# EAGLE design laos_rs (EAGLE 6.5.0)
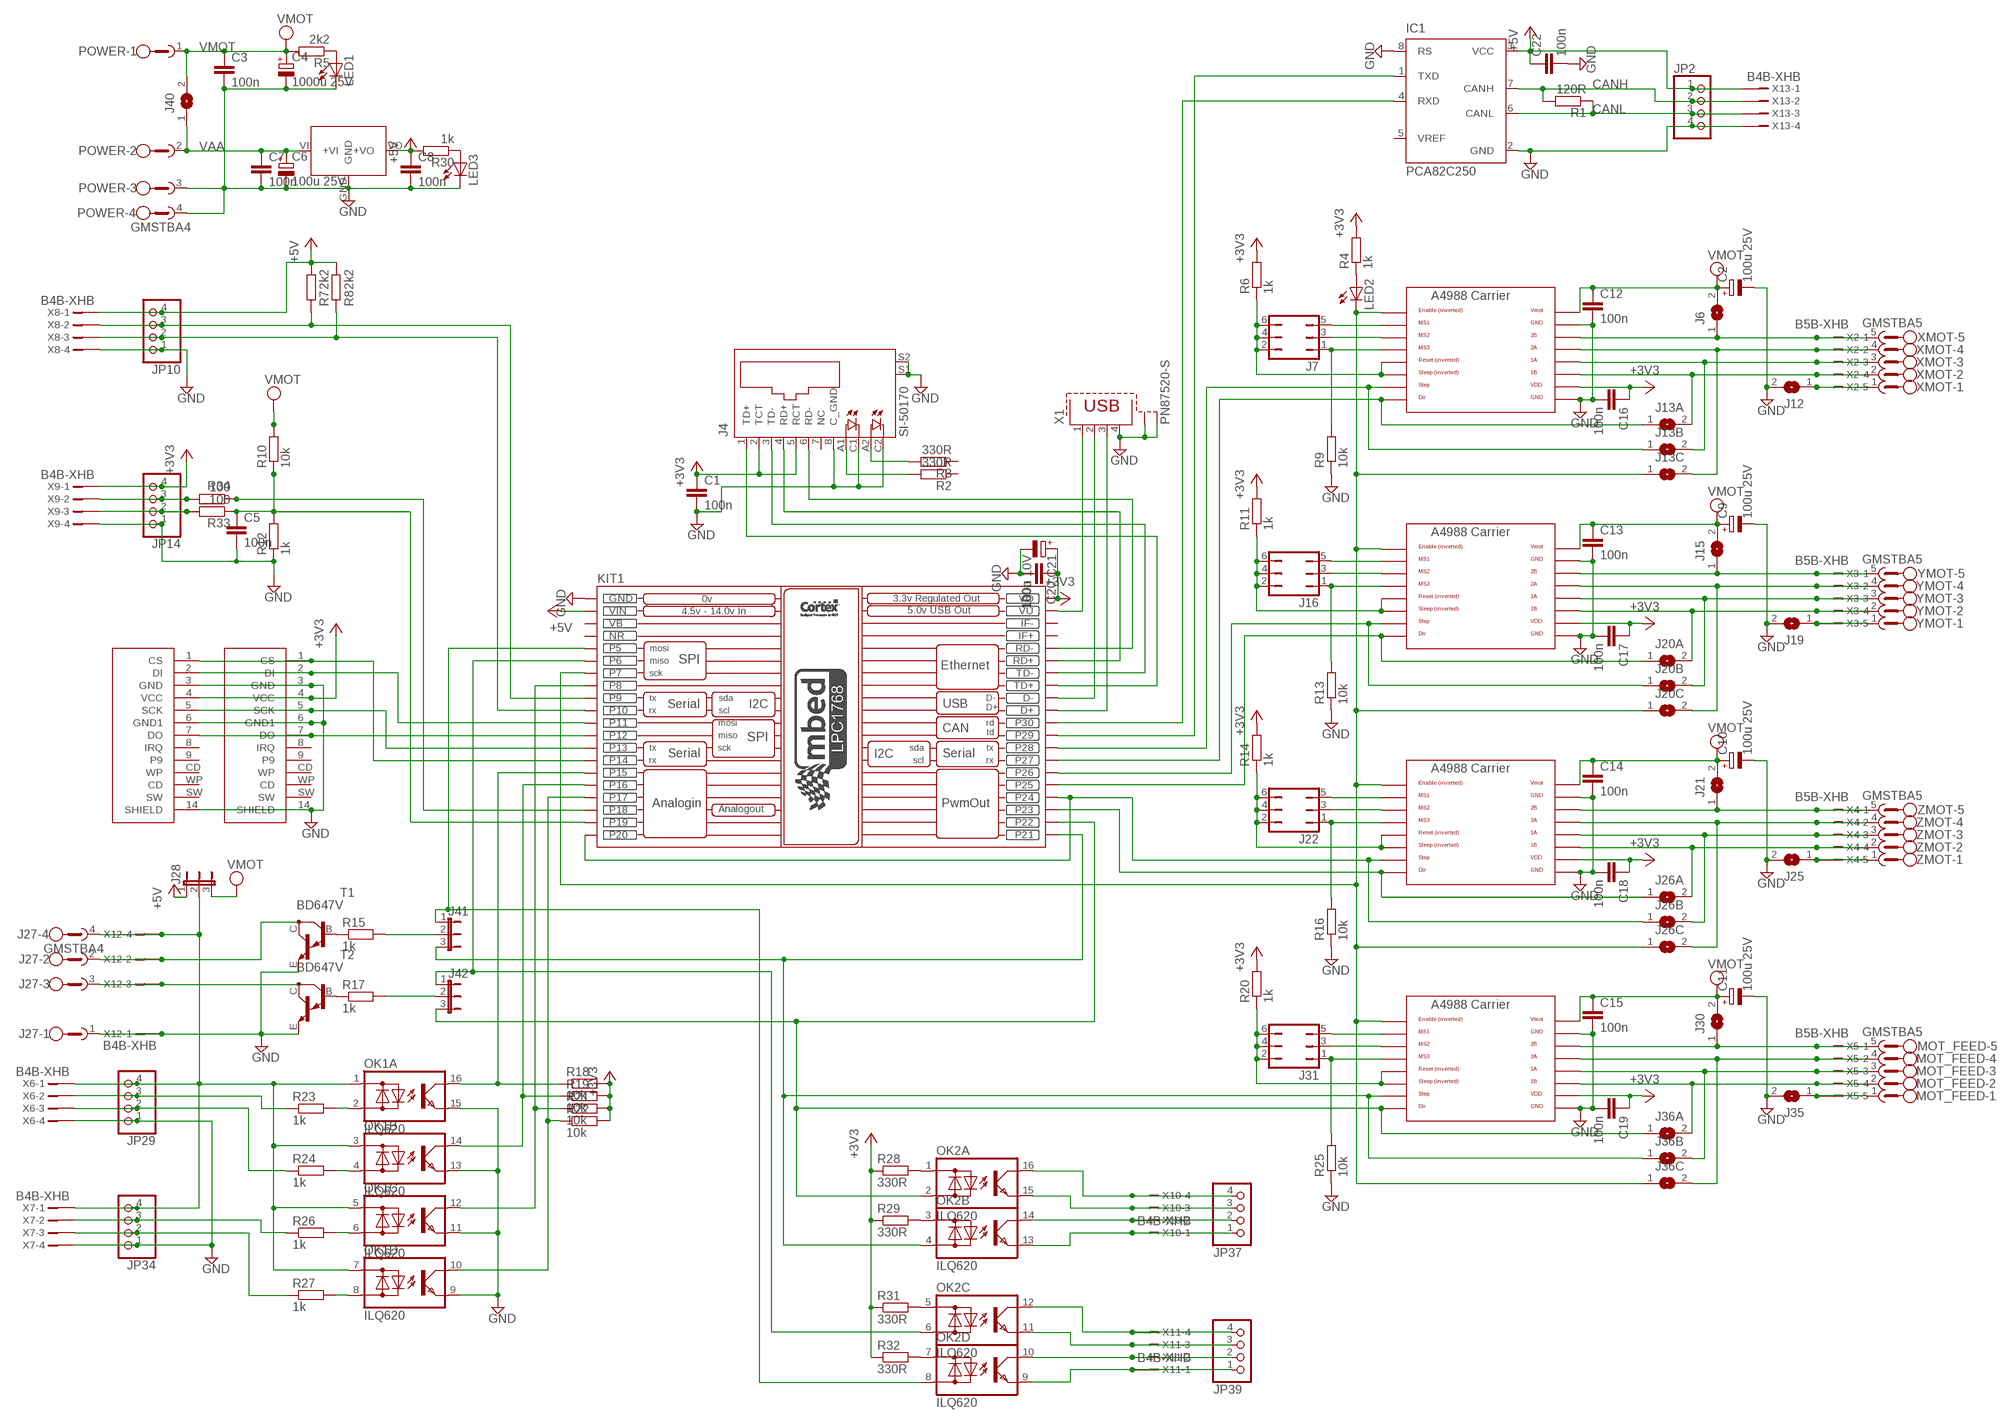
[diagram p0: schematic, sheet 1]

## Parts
C1  100n  C-EU025_050-025X075  [C025_050-025X075]
C2  100u 25V  CPOL-EUE5-8.5  [E5-8,5]
C3  100n  C-EU025_050-025X075  [C025_050-025X075]
C4  1000u 25V  CPOL-EUE5-13  [E5-13]
C5  100n  C-EU050-025X075  [C050-025X075]
C6  100u 25V  CPOL-EUE5-10.5  [E5-10,5]
C7  100n  C-EU025_050-025X075  [C025_050-025X075]
C8  100n  C-EU025_050-025X075  [C025_050-025X075]
C9  100u 25V  CPOL-EUE5-8.5  [E5-8,5]
C10  100u 25V  CPOL-EUE5-8.5  [E5-8,5]
C11  100u 25V  CPOL-EUE5-8.5  [E5-8,5]
C12  100n  C-EU025_050-025X075  [C025_050-025X075]
C13  100n  C-EU025_050-025X075  [C025_050-025X075]
C14  100n  C-EU025_050-025X075  [C025_050-025X075]
C15  100n  C-EU025_050-025X075  [C025_050-025X075]
C16  100n  C-EU025_050-025X075  [C025_050-025X075]
C17  100n  C-EU025_050-025X075  [C025_050-025X075]
C18  100n  C-EU025_050-025X075  [C025_050-025X075]
C19  100n  C-EU025_050-025X075  [C025_050-025X075]
C20  100n  C-EU025_050-025X075  [C025_050-025X075]
C21  100u 10V  CPOL-EUE5-8.5  [E5-8,5]
C22  100n  C-EU025_050-025X075  [C025_050-025X075]
IC1  PCA82C250  [DIL08]
J4  SI-50170  [SI-50170]
J6  SJ  [SJ]
J7  JP3Q  [JP3Q]
J12  SJ  [SJ]
J13A  SJ  [SJ]
J13B  SJ  [SJ]
J13C  SJ  [SJ]
J15  SJ  [SJ]
J16  JP3Q  [JP3Q]
J19  SJ  [SJ]
J20A  SJ  [SJ]
J20B  SJ  [SJ]
J20C  SJ  [SJ]
J21  SJ  [SJ]
J22  JP3Q  [JP3Q]
J25  SJ  [SJ]
J26A  SJ  [SJ]
J26B  SJ  [SJ]
J26C  SJ  [SJ]
J27  GMSTBA4  [GMSTBA4]
J28  JP2E  [JP2]
J30  SJ  [SJ]
J31  JP3Q  [JP3Q]
J35  SJ  [SJ]
J36A  SJ  [SJ]
J36B  SJ  [SJ]
J36C  SJ  [SJ]
J40  SJW  [SJW]
J41  JP2E  [JP2]
J42  JP2E  [JP2]
JP2  PINHD-1X04_2.54  [1X04]
JP10  PINHD-1X04_2.54  [1X04]
JP14  PINHD-1X04_2.54  [1X04]
JP29  PINHD-1X04_2.54  [1X04]
JP34  PINHD-1X04_2.54  [1X04]
JP37  PINHD-1X04_2.54  [1X04]
JP39  PINHD-1X04_2.54  [1X04]
KIT1  MBED_NXP_LPC1768  [MBED-KIT]
LED1  LED3MM  [LED3MM]
LED2  LED3MM  [LED3MM]
LED3  LED3MM  [LED3MM]
MOT_FEED  GMSTBA5  [GMSTBA5]
OK1  ILQ620  [DIL16]
OK2  ILQ620  [DIL16]
POWER  GMSTBA4  [GMSTBA4]
R1  120R  R-EU0207/2V  [0207/2V]
R2  330R  R-EU0207/10  [0207/10]
R3  330R  R-EU0207/10  [0207/10]
R4  1k  R-EU0207/10  [0207/10]
R5  2k2  R-EU0207/10  [0207/10]
R6  1k  R-EU0207/10  [0207/10]
R7  2k2  R-EU0207/10  [0207/10]
R8  2k2  R-EU0207/10  [0207/10]
R9  10k  R-EU0207/10  [0207/10]
R10  10k  R-EU0207/10  [0207/10]
R11  1k  R-EU0207/10  [0207/10]
R12  1k  R-EU0207/10  [0207/10]
R13  10k  R-EU0207/10  [0207/10]
R14  1k  R-EU0207/10  [0207/10]
R15  1k  R-EU0207/10  [0207/10]
R16  10k  R-EU0207/10  [0207/10]
R17  1k  R-EU0207/10  [0207/10]
R18  10k  R-EU0207/10  [0207/10]
R19  10k  R-EU0207/10  [0207/10]
R20  1k  R-EU0207/10  [0207/10]
R21  10k  R-EU0207/10  [0207/10]
R22  10k  R-EU0207/10  [0207/10]
R23  1k  R-EU0207/10  [0207/10]
R24  1k  R-EU0207/10  [0207/10]
R25  10k  R-EU0207/10  [0207/10]
R26  1k  R-EU0207/10  [0207/10]
R27  1k  R-EU0207/10  [0207/10]
R28  330R  R-EU0207/10  [0207/10]
R29  330R  R-EU0207/10  [0207/10]
R30  1k  R-EU0207/10  [0207/10]
R31  330R  R-EU0207/10  [0207/10]
R32  330R  R-EU0207/10  [0207/10]
R33  100  R-EU0207/10  [0207/10]
R34  100  R-EU0207/10  [0207/10]
T1  BD647V  [TO220AV]
T2  BD647V  [TO220AV]
U4  SD_CARD_SOCKETSD  [SD-MMC_SOCKET-PP]
U11  SD_CARD_SOCKETSD  [SD-MMC_SOCKET-PP]
U$1  POLOLU_A4983CARRIER  [A4988BREAKOUT]
U$2  POLOLU_A4983CARRIER  [A4988BREAKOUT]
U$3  POLOLU_A4983CARRIER  [A4988BREAKOUT]
U$5  R-78B-  [R-78B**-*]
U$6  POLOLU_A4983CARRIER  [A4988BREAKOUT]
X1  PN87520-S  [PN87520-S]
X2  B5B-XHB  [B5B-XH]
X3  B5B-XHB  [B5B-XH]
X4  B5B-XHB  [B5B-XH]
X5  B5B-XHB  [B5B-XH]
X6  B4B-XHB  [B4B-XH]
X7  B4B-XHB  [B4B-XH]
X8  B4B-XHB  [B4B-XH]
X9  B4B-XHB  [B4B-XH]
X10  B4B-XHB  [B4B-XH]
X11  B4B-XHB  [B4B-XH]
X12  B4B-XHB  [B4B-XH]
X13  B4B-XHB  [B4B-XH]
XMOT  GMSTBA5  [GMSTBA5]
YMOT  GMSTBA5  [GMSTBA5]
ZMOT  GMSTBA5  [GMSTBA5]

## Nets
+3V3: C1.1 C16.1 C17.1 C18.1 C19.1 C20.1 C21.+ J4.2(TCT) J4.5(RCT) JP14.4 KIT1.VOUT(VO) R4.2 R6.2 R11.2 R14.2 R18.2 R19.2 R20.2 R21.2 R22.2 R28.1 R29.1 R31.1 R32.1 U4.4(VCC) U11.4(VCC) U$1.VDD U$2.VDD U$3.VDD U$6.VDD X9.1
+5V: C8.1 C22.1 IC1.3(VCC) J28.1 JP2.1 JP10.4 KIT1.VIN R7.2 R8.2 R30.2 U$5.VO(+VO) X8.1 X13.1
/ENABLE: J13C.1 J20C.1 J26C.1 J36C.1 KIT1.7 LED2.K(C) U$1.EN U$2.EN U$3.EN U$6.EN
ANALOG_IN: C5.1 KIT1.19 R10.1 R12.2 R33.1
ANALOG_OUT: KIT1.18 R34.1
AUX1: J27.2 T1.C X12.2
AUX2: J27.3 T2.C X12.3
CANH: IC1.7(CANH) JP2.2 R1.2 X13.2
CANL: IC1.6(CANL) JP2.3 R1.1 X13.3
D+: KIT1.D+ X1.3
D-: KIT1.D- X1.2
DIR_FEED: J36A.1 J42.3 KIT1.22 OK2.2(A:AC2) U$6.DIR
DIR_X: J13A.1 KIT1.27 U$1.DIR
DIR_Y: J20A.1 KIT1.25 U$2.DIR
DIR_Z: J26A.1 KIT1.23 U$3.DIR
EXHAUST_ENABLE_C: JP37.4 OK2.16(A:C) X10.4
EXHAUST_ENABLE_E: JP37.3 OK2.15(A:E) X10.3
GND: C1.2 C1.3 C2.- C3.2 C3.3 C4.- C5.2 C6.- C7.2 C7.3 C8.2 C8.3 C9.- C10.- C11.- C12.2 C12.3 C13.2 C13.3 C14.2 C14.3 C15.2 C15.3 C16.2 C16.3 C17.2 C17.3 C18.2 C18.3 C19.2 C19.3 C20.2 C20.3 C21.- C22.2 C22.3 IC1.2(GND) IC1.8(RS) J4.8(C_GND) J4.C1(C) J4.C2(C1) J4.S1 J4.S2 J12.2 J19.2 J25.2 J27.1 J35.2 JP2.4 JP10.1 JP14.1 JP29.1 JP34.1 KIT1.GND LED1.K(C) LED3.K(C) OK1.9(D:E) OK1.11(C:E) OK1.13(B:E) OK1.15(A:E) POWER.3 POWER.4 R9.1 R12.1 R13.1 R16.1 R25.1 T1.E T2.E U4.3(GND) U4.6(GND1) U4.14(SHIELD) U11.3(GND) U11.6(GND1) U11.14(SHIELD) U$1.GND U$1.GND@0(GND) U$2.GND U$2.GND@0(GND) U$3.GND U$3.GND@0(GND) U$5.GND U$6.GND U$6.GND@0(GND) X1.4 X1.S1 X1.S2 X6.4 X7.4 X8.4 X9.4 X12.1 X13.4
LASER_ENABLE_C: JP37.2 OK2.14(B:C) X10.2
LASER_ENABLE_E: JP37.1 OK2.13(B:E) X10.1
LASER_ON: J41.1 KIT1.5 OK2.8(D:AC2)
LASER_ON_E: JP39.1 OK2.9(D:E) X11.1
LASER_PWM: J42.1 KIT1.6 OK2.6(C:AC2)
LASER_PWM_C: JP39.4 OK2.12(C:C) X11.4
LASER_PWM_E: JP39.3 OK2.11(C:E) X11.3
N$1: J15.1 U$2.2B X3.1 YMOT.5
N$2: J20C.2 U$2.2A X3.2 YMOT.4
N$3: J20B.2 U$2.1A X3.3 YMOT.3
N$4: J20A.2 U$2.1B X3.4 YMOT.2
N$5: J6.1 U$1.2B X2.1 XMOT.5
N$6: J13C.2 U$1.2A X2.2 XMOT.4
N$7: J13B.2 U$1.1A X2.3 XMOT.3
N$8: J13A.2 U$1.1B X2.4 XMOT.2
N$9: J21.1 U$3.2B X4.1 ZMOT.5
N$10: J26C.2 U$3.2A X4.2 ZMOT.4
N$11: J26B.2 U$3.1A X4.3 ZMOT.3
N$12: J26A.2 U$3.1B X4.4 ZMOT.2
N$13: OK2.1(A:AC1) R28.2
N$14: OK2.3(B:AC1) R29.2
N$15: OK2.5(C:AC1) R31.2
N$16: OK2.7(D:AC1) R32.2
N$17: OK1.2(A:AC2) R23.2
N$18: OK1.4(B:AC2) R24.2
N$19: OK1.6(C:AC2) R26.2
N$20: OK1.8(D:AC2) R27.2
N$22: J12.1 X2.5 XMOT.1
N$23: J19.1 X3.5 YMOT.1
N$24: J25.1 X4.5 ZMOT.1
N$28: KIT1.VU X1.1
N$29: J7.2 J7.4 J7.6 R6.1 U$1.RST U$1.SLP(SLEEP)
N$30: J7.5 U$1.MS1
N$31: J7.3 U$1.MS2
N$32: J7.1 R9.2 U$1.MS3
N$34: J16.2 J16.4 J16.6 R11.1 U$2.RST U$2.SLP(SLEEP)
N$35: J16.5 U$2.MS1
N$36: J16.3 U$2.MS2
N$37: J16.1 R13.2 U$2.MS3
N$39: J22.2 J22.4 J22.6 R14.1 U$3.RST U$3.SLP(SLEEP)
N$40: J22.5 U$3.MS1
N$41: J22.3 U$3.MS2
N$42: J22.1 R16.2 U$3.MS3
N$49: JP14.2 R33.2 X9.3
N$55: J35.1 MOT_FEED.1 X5.5
N$57: J4.A1(A) R2.2
N$60: JP14.3 R34.2 X9.2
N$64: R15.1 T1.B
N$65: R17.1 T2.B
N$68: JP39.2 OK2.10(D:C) X11.2
N$75: J4.A2(A1) R3.2
N$76: J41.2 R15.2
N$77: J42.2 R17.2
N$82: J30.1 MOT_FEED.5 U$6.2B X5.1
N$83: J36C.2 MOT_FEED.4 U$6.2A X5.2
N$84: J36B.2 MOT_FEED.3 U$6.1A X5.3
N$85: J36A.2 MOT_FEED.2 U$6.1B X5.4
N$86: LED3.A R30.1
N$90: J31.2 J31.4 J31.6 R20.1 U$6.RST U$6.SLP(SLEEP)
N$91: J31.5 U$6.MS1
N$92: J31.3 U$6.MS2
N$93: J31.1 R25.2 U$6.MS3
N$105: LED1.A R5.1
N$106: LED2.A R4.1
P8: KIT1.8 OK1.12(C:C) R21.1
P11: KIT1.11 U4.2(DI) U11.2(DI)
P12: KIT1.12 U4.7(DO) U11.7(DO)
P13: KIT1.13 U4.5(SCK) U11.5(SCK)
P14: KIT1.14 U4.1(CS) U11.1(CS)
P15: KIT1.15 OK1.16(A:C) R18.1
P16: KIT1.16 OK1.14(B:C) R19.1
P17: KIT1.17 OK1.10(D:C) R22.1
P29: IC1.1(TXD) KIT1.29
P30: IC1.4(RXD) KIT1.30
RD+: J4.4(RD+) KIT1.RD+
RD-: J4.6(RD-) KIT1.RD-
SCL: JP10.2 KIT1.10 R8.1 X8.3
SDA: JP10.3 KIT1.9 R7.1 X8.2
STEP_FEED: J36B.1 J41.3 KIT1.21 OK2.4(B:AC2) U$6.STEP
STEP_X: J13B.1 KIT1.28 U$1.STEP
STEP_Y: J20B.1 KIT1.26 U$2.STEP
STEP_Z: J26B.1 KIT1.20 KIT1.24 U$3.STEP
TD+: J4.1(TD+) KIT1.TD+
TD-: J4.3(TD-) KIT1.TD-
V_ENDSTOP: J27.4 J28.2 JP29.4 JP34.4 OK1.1(A:AC1) OK1.3(B:AC1) OK1.5(C:AC1) OK1.7(D:AC1) X6.1 X7.1 X12.4
VAA: C6.+ C7.1 J40.1 POWER.2 U$5.VI(+VI)
VMOT: C2.+ C3.1 C4.+ C9.+ C10.+ C11.+ C12.1 C13.1 C14.1 C15.1 J6.2 J15.2 J21.2 J28.3 J30.2 J40.2 POWER.1 R5.2 R10.2 U$1.VMOT U$2.VMOT U$3.VMOT U$6.VMOT
X_HOME: JP29.3 R23.1 X6.2
Y_HOME: JP29.2 R24.1 X6.3
Z+: JP34.3 R26.1 X7.2
Z-: JP34.2 R27.1 X7.3
Unconnected: IC1.5(VREF) J4.7(NC) KIT1.IF+ KIT1.IF- R2.1 R3.1 U4.8(IRQ) U4.9 U4.CD(WP) U4.SW U4.WP(CD) U11.8(IRQ) U11.9 U11.CD(WP) U11.SW U11.WP(CD)

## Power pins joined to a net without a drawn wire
NR: KIT1.NR
VB: KIT1.VB

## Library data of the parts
C1 C3 C5 C7 C8 C12-C20 C22 = rcl:C-EU: CAPACITOR, European symbol
C2 C4 C6 C9-C11 C21 = rcl:CPOL-EU: POLARIZED CAPACITOR, European symbol
IC1 = micro-philips:PCA82C250: CAN CONTROLLER INTERFACE
J4 = con-rj45-v3:SI-50170: Ethernet Connector MagJack (R) Source: www.stewartconnector.com .. si-50170.pdf
J6 J12 J13A J13B J13C J15 J19 J20A J20B J20C J21 J25 J26A J26B J26C J30 J35 J36A J36B J36C J40 = jumper:SJ: SMD solder JUMPER
J7 J16 J22 J31 = jumper:JP3Q: JUMPER
J27 POWER = con-phoenix-762:GMSTBA4: PHOENIX; MF: FARNELL; MPN: 1757268; OC_FARNELL: 3705195; OC_NEWARK: 71C4163
J28 J41 J42 = jumper:JP2E: JUMPER
JP2 JP10 JP14 JP29 JP34 JP37 JP39 = con-pinhead-2:PINHD-1X04: PIN HEADER
KIT1 = MBED_v2.1:MBED_NXP_LPC1768: Mbed LPC1768 - ARM CORTEX v2.1 * Schematic symbol is now placed in eagles's default raster. *The pads diameter are suitable for routing between mbed pins * mbed pads are 0.8 mm drill diameter. --------------------------------------------- Created by: Mohamed Yousry *Alexandria, Egypt *Email: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
LED1-LED3 = led:LED: LED
MOT_FEED XMOT YMOT ZMOT = con-phoenix-762:GMSTBA5: PHOENIX
OK1 OK2 = optocoupler-3:ILQ620: SIEMENS OPTO COUPLER
R1-R34 = rcl:R-EU: RESISTOR, European symbol
T1 T2 = transistor-power:BD647: NPN BIPOLAR DARLINGTON TRANSISTOR
U4 U11 = SparkFun:SD_CARD_SOCKET: SD/MMC Socket Media socket for SD and MMC cards. Push-push type. Schematic element and footprint production proven. Spark Fun Electronics SKU : PRT-00136
U$1-U$3 U$6 = RepRapjr:POLOLU_A4983CARRIER
U$5 = v-reg_recom:R-78B**-*: RECOM R-78B**-* switching regulator (78xx compatible)
X1 = con-berg-usb:PN87520-S: BERG USB A connector (shielded)
X2-X5 = con-jst:B5B-XH: XH CONNECTOR 2.5 mm, 5 pin 1 row Source: http://www.jst.com .. eXH.pdf
X6-X13 = con-jst:B4B-XH: XH CONNECTOR 2.5 mm, 4 pin 1 row Source: http://www.jst.com .. eXH.pdf

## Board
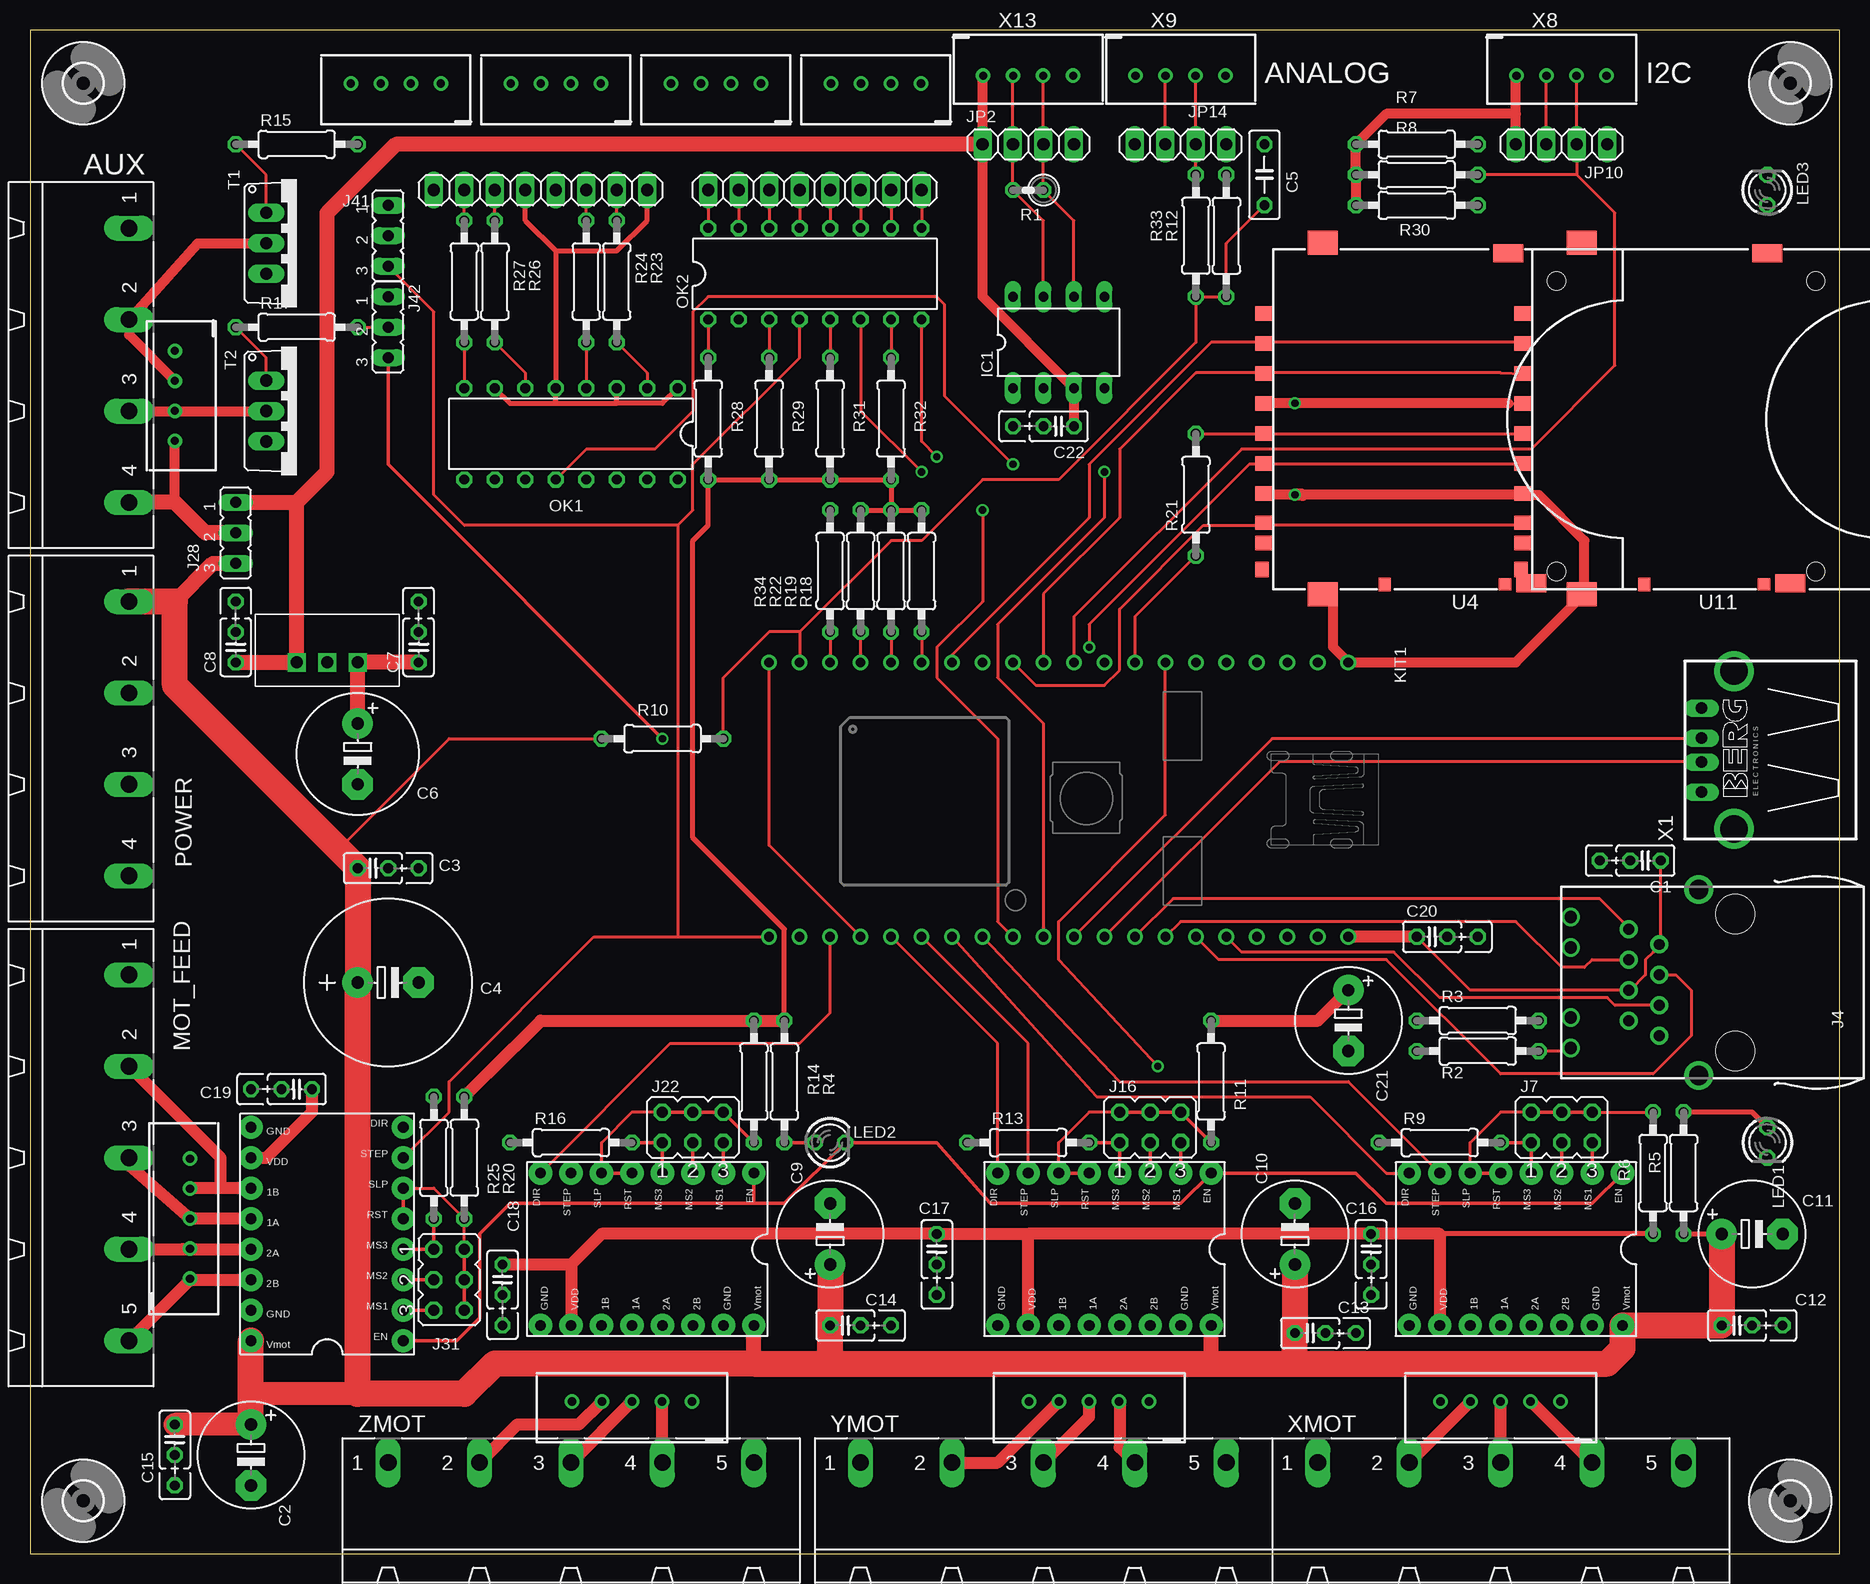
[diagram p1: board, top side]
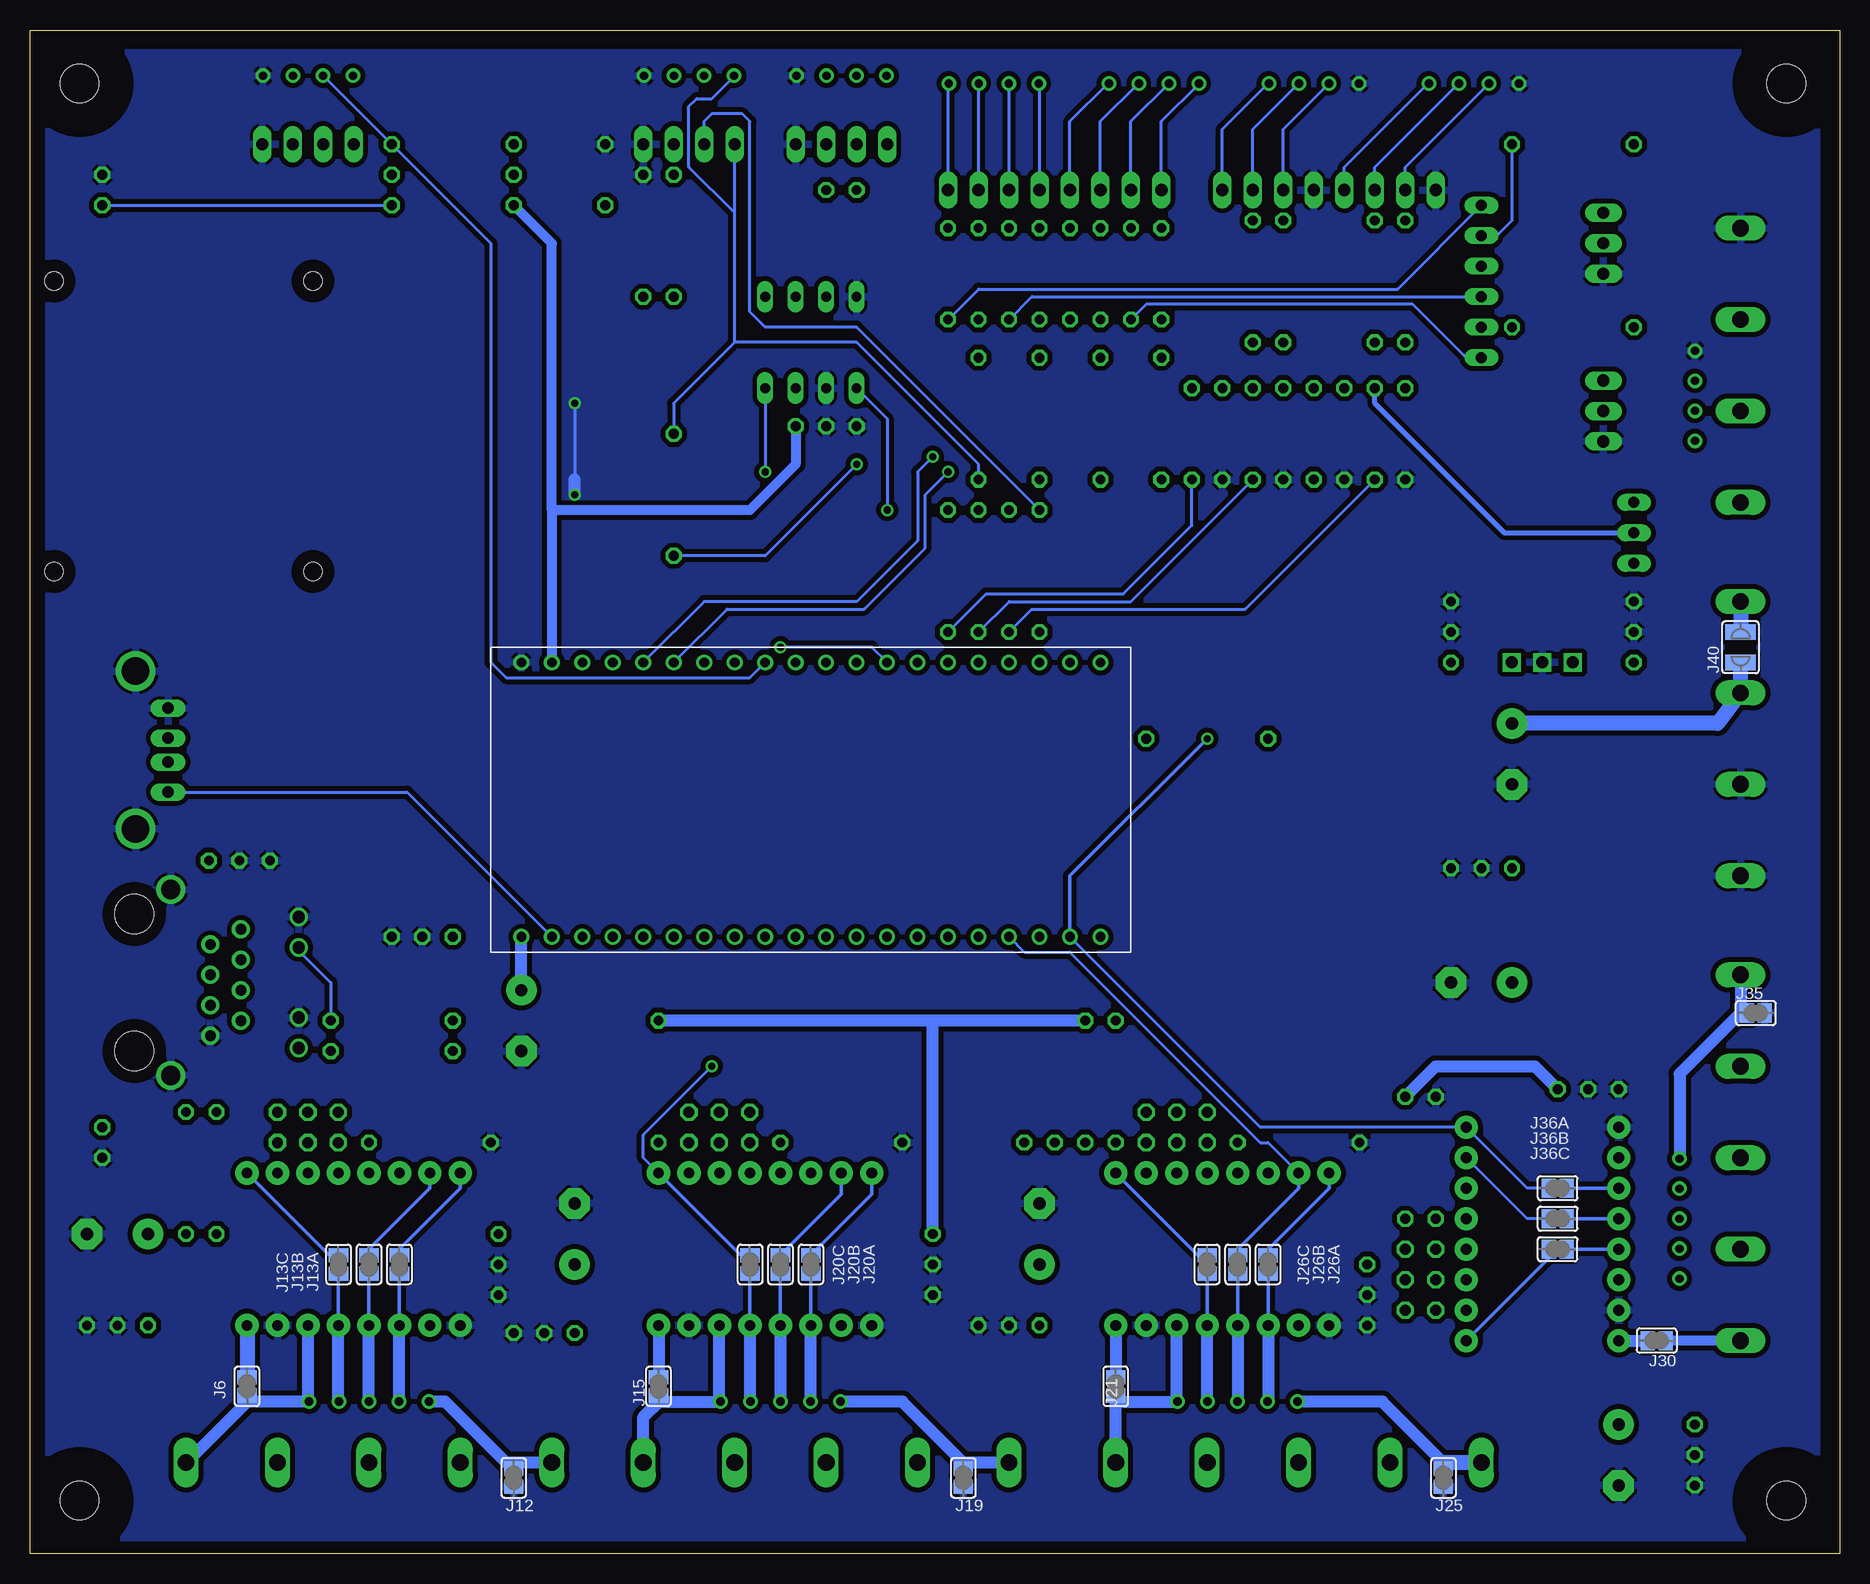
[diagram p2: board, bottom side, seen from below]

Size 150.8 x 126.98 mm. Coordinates in mm from the lower left corner, seen from the top.
Outline: 0,126.98 0,0 150.8,0 150.8,126.98 0,126.98
Copper layers (1*16): Top 0.035mm / dielectric 1.5mm / Bottom 0.035mm
Design rules "default": minimum track width 10mil, minimum drill 0.6mm, track to track 8mil, track to pad 8mil, pad to pad 8mil, via to via 8mil, smd to smd 8mil, copper to edge 40mil, drill to drill 8mil, minimum pad ring 10mil, minimum via ring 8mil, stop-mask expansion 4mil, vias tented up to drill 0mil, thermal gap 10mil

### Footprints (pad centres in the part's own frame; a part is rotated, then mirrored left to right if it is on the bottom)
C025_050-025X075 = drill 0.813 octagon: 1 -1.27,0; 2 1.27,0; 3 3.81,0
E5-8,5 = drill 1.016 pad 2.54: + -2.54,0 | drill 1.016 pad 2.54 octagon: - 2.54,0
E5-13 = drill 1.016 pad 2.54: + -2.54,0 | drill 1.016 pad 2.54 octagon: - 2.54,0
C050-025X075 = drill 0.813 octagon: 1 -2.54,0; 2 2.54,0
E5-10,5 = drill 1.016 pad 2.54: + -2.54,0 | drill 1.016 pad 2.54 octagon: - 2.54,0
DIL08 = drill 0.813 long: 1 -3.81,-3.81; 2 -1.27,-3.81; 3 1.27,-3.81; 4 3.81,-3.81; 5 3.81,3.81; 6 1.27,3.81; 7 -1.27,3.81; 8 -3.81,3.81
SI-50170 = drill 0.9 pad 1.5: 1 4.445,5.842; 2 3.175,3.302; 3 1.905,5.842; 4 0.635,3.302; 5 -0.635,5.842; 6 -1.905,3.302; 7 -3.175,5.842; 8 -4.445,3.302 | drill 1.016 pad 1.5: A1 -5.461,10.668; A2 2.921,10.668; C1 -2.921,10.668; C2 5.461,10.668 | drill 1.6 pad 2.2: S1 -7.747,0; S2 7.747,0 | hole 3.251: -5.715,-3.048; 5.715,-3.048
SJ = smd 1.168 x 1.6: 1 -0.762,0; 2 0.762,0
JP3Q = drill 0.914 octagon: 1 -2.54,-1.27; 2 -2.54,1.27; 3 0,-1.27; 4 0,1.27; 5 2.54,-1.27; 6 2.54,1.27
GMSTBA4 = drill 1.397 long: 1 -11.43,5.08; 2 -3.81,5.08; 3 3.81,5.08; 4 11.43,5.08
JP2 = drill 0.914 long: 1 -2.54,0; 2 0,0; 3 2.54,0
SJW = smd 1.27 x 2.54: 1 -1.27,0; 2 1.27,0
1X04 = drill 1.016 long: 1 -3.81,0; 2 -1.27,0; 3 1.27,0; 4 3.81,0
MBED-KIT = drill 0.8: 5 -11.43,13.97; 6 -11.43,11.43; 7 -11.43,8.89; 8 -11.43,6.35; 9 -11.43,3.81; 10 -11.43,1.27; 11 -11.43,-1.27; 12 -11.43,-3.81; 13 -11.43,-6.35; 14 -11.43,-8.89; 15 -11.43,-11.43; 16 -11.43,-13.97; 17 -11.43,-16.51; 18 -11.43,-19.05; 19 -11.43,-21.59; 20 -11.43,-24.13; 21 11.43,-24.13; 22 11.43,-21.59; 23 11.43,-19.05; 24 11.43,-16.51; 25 11.43,-13.97; 26 11.43,-11.43; 27 11.43,-8.89; 28 11.43,-6.35; 29 11.43,-3.81; 30 11.43,-1.27; D+ 11.43,1.27; D- 11.43,3.81; GND -11.43,24.13; IF+ 11.43,16.51; IF- 11.43,19.05; NR -11.43,16.51; RD+ 11.43,11.43; RD- 11.43,13.97; TD+ 11.43,6.35; TD- 11.43,8.89; VB -11.43,19.05; VIN -11.43,21.59; VOUT 11.43,24.13; VU 11.43,21.59
LED3MM = drill 0.813 octagon: A -1.27,0; K 1.27,0
GMSTBA5 = drill 1.397 long: 1 -15.24,5.08; 2 -7.62,5.08; 3 0,5.08; 4 7.62,5.08; 5 15.24,5.08
DIL16 = drill 0.813 octagon: 1 -8.89,-3.81; 2 -6.35,-3.81; 3 -3.81,-3.81; 4 -1.27,-3.81; 5 1.27,-3.81; 6 3.81,-3.81; 7 6.35,-3.81; 8 8.89,-3.81; 9 8.89,3.81; 10 6.35,3.81; 11 3.81,3.81; 12 1.27,3.81; 13 -1.27,3.81; 14 -3.81,3.81; 15 -6.35,3.81; 16 -8.89,3.81
0207/2V = drill 0.813 octagon: 1 -1.27,0; 2 1.27,0
0207/10 = drill 0.813 octagon: 1 -5.08,0; 2 5.08,0
TO220AV = drill 1.016 long: B -2.54,-2.54; C 0,-2.54; E 2.54,-2.54
SD-MMC_SOCKET-PP = smd 1.2 x 1.5: 1 6.88,29.85; 2 4.38,29.85; 3 1.88,29.85; 4 -0.62,29.85; 5 -3.12,29.85; 6 -5.62,29.85; 7 -8.04,29.85; 8 -9.728,29.87; 9 9.38,29.85 | smd 1.5 x 2.5: 12 -13.1,7.6; 13 14.402,9.525 | smd 2 x 2.5: 14 -14,25; 15 15.3,25 | smd 1.15 x 1: CD -13.18,19.8 | smd 1.3 x 1.1: SW -11.938,30.048 | smd 1 x 1.05: WP -13.18,9.8 | hole 1.5: -12.1,5.5; 12.1,5.5
A4988BREAKOUT = drill 0.9 pad 1.93: 1A 8.89,1.27; 1B 11.43,1.27; 2A 6.35,1.27; 2B 3.81,1.27; DIR 16.51,-11.43; EN -1.27,-11.43; GND 16.51,1.27; GND@0 1.27,1.27; MS1 1.27,-11.43; MS2 3.81,-11.43; MS3 6.35,-11.43; RST 8.89,-11.43; SLP 11.43,-11.43; STEP 13.97,-11.43; VDD 13.97,1.27; VMOT -1.27,1.27
R-78B**-* = drill 1 square: GND 0,0; VI -2.54,0; VO 2.54,0
3,2 = hole 3.2: 0,0
PN87520-S = drill 0.95 long: 1 -3.5,2.71; 2 -1,2.71; 3 1,2.71; 4 3.5,2.71 | drill 2.3 pad 2.9: S1 -6.57,0; S2 6.57,0
B5B-XH = drill 0.7 pad 1.1: 1 -5,0; 2 -2.5,0; 3 0,0; 4 2.5,0; 5 5,0
B4B-XH = drill 0.7 pad 1.1: 1 -3.75,0; 2 -1.25,0; 3 1.25,0; 4 3.75,0

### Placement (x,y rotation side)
C1  134.62,57.76 180 top
C2  18.41,8.24 270 top
C3  28.57,57.13 0 top
C4  29.84,47.6 0 top
C5  102.87,114.92 90 top
C6  27.3,66.66 270 top
C7  32.38,75.55 90 top
C8  17.14,75.55 90 top
C9  66.67,26.65 90 top
C10  105.41,26.65 90 top
C11  143.51,26.65 0 top
C12  142.24,19.03 0 top
C13  106.68,18.39 0 top
C14  67.94,19.03 0 top
C15  12.06,9.51 270 top
C16  111.76,25.38 270 top
C17  75.56,25.38 270 top
C18  39.37,22.84 270 top
C19  22.23,38.71 180 top
C20  116.84,51.41 0 top
C21  109.86,44.43 270 top
C22  85.72,93.96 180 top
IC1  85.72,100.95 0 top
J4  139.06,47.6 90 top
J6  132.72,13.95 90 bottom
J7  127.64,35.54 0 top
J12  110.49,6.33 270 bottom
J13A  120.02,24.11 270 bottom
J13B  122.56,24.11 270 bottom
J13C  125.09,24.11 270 bottom
J15  98.42,13.95 90 bottom
J16  93.34,35.54 0 top
J19  73.03,6.33 270 bottom
J20A  85.72,24.11 270 bottom
J20B  88.27,24.11 270 bottom
J20C  90.81,24.11 270 bottom
J21  60.33,13.95 90 bottom
J22  55.24,35.54 0 top
J25  33.02,6.33 270 bottom
J26A  47.62,24.11 270 bottom
J26B  50.16,24.11 270 bottom
J26C  52.7,24.11 270 bottom
J27  3.17,99.04 270 top
J28  17.14,85.07 270 top
J30  15.24,17.76 180 bottom
J31  34.92,22.84 270 top
J35  6.99,45.06 0 bottom
J36A  23.5,30.46 0 bottom
J36B  23.5,27.92 0 bottom
J36C  23.5,25.38 0 bottom
J40  8.26,75.55 90 bottom
J41  29.84,109.84 270 top
J42  29.84,102.22 270 top
JP2  83.19,117.45 0 top
JP10  127.64,117.45 180 top
JP14  95.89,117.45 180 top
JP29  47.62,113.65 0 top
JP34  37.47,113.65 0 top
JP37  60.33,113.65 180 top
JP39  70.48,113.65 180 top
KIT1  85.72,62.84 270 top
LED1  144.78,34.27 270 top
LED2  66.67,34.27 0 top
LED3  144.78,113.65 90 top
MOT_FEED  3.17,33 270 top
OK1  45.09,93.33 180 top
OK2  65.41,106.66 0 top
POWER  3.17,67.92 270 top
R1  83.19,113.65 180 top
R2  120.65,41.89 0 top
R3  120.65,44.43 0 top
R4  62.87,39.35 90 top
R5  137.79,31.73 270 top
R6  135.25,31.73 270 top
R7  115.57,117.45 180 top
R8  115.57,114.92 180 top
R9  117.47,34.27 0 top
R10  52.7,67.92 180 top
R11  98.42,39.35 90 top
R12  99.69,109.84 270 top
R13  83.19,34.27 0 top
R14  60.33,39.35 90 top
R15  22.23,117.45 0 top
R16  45.09,34.27 0 top
R17  22.23,102.22 0 top
R18  74.3,81.9 90 top
R19  71.75,81.9 90 top
R20  36.2,33 90 top
R21  97.16,88.25 90 top
R22  69.22,81.9 90 top
R23  48.9,106.03 270 top
R24  46.35,106.03 270 top
R25  33.66,33 270 top
R26  38.73,106.03 270 top
R27  36.2,106.03 270 top
R28  56.52,94.59 90 top
R29  61.59,94.59 90 top
R30  115.57,112.38 180 top
R31  66.67,94.59 90 top
R32  71.75,94.59 90 top
R33  97.16,109.84 90 top
R34  66.67,81.9 90 top
T1  22.23,109.2 270 top
T2  22.23,95.23 270 top
U4  132.72,93.96 90 top
U11  154.31,93.96 90 top
U$1  131.44,20.3 180 top
U$2  97.16,20.3 180 top
U$3  59.05,20.3 180 top
U$5  R-78B*-*  [R-78B**-*]  24.77,74.28 180 top
U$6  19.68,19.03 90 top
U$7  [3,2]  4.45,4.43 0 top
U$8  [3,2]  146.69,4.43 0 top
U$9  [3,2]  146.69,122.54 0 top
U$10  [3,2]  4.45,122.54 0 top
X1  142,66.98 90 top
X2  122.56,12.68 180 top
X3  88.27,12.68 180 top
X4  50.16,12.68 180 top
X5  13.34,27.92 90 top
X6  43.81,122.54 180 top
X7  30.48,122.54 180 top
X8  127.64,123.17 0 top
X9  95.89,123.17 0 top
X10  57.15,122.54 180 top
X11  70.48,122.54 180 top
X12  12.06,96.5 270 top
X13  83.19,123.17 0 top
XMOT  122.56,2.52 0 top
YMOT  84.45,2.52 0 top
ZMOT  45.09,2.52 0 top

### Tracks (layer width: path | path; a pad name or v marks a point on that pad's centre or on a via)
+3V3
  Top 0.254: C1.1 135.89,50.78 J4.2 135.25,50.14 134.62,49.51 134.62,48.24 133.35,46.97 J4.5 120.02,46.97 C20.1 | R21.2 102.87,93.33 U4.4 103.5,93.33 122.56,93.33 U11.4
  Top 0.406: R6.2 117.47,26.65 | R22.2 R19.2 | R19.2 R18.2 | R4.2 62.87,52.05 55.24,59.67 55.24,84.44 56.52,85.7 R28.1 R29.1 R31.1 R32.1 R19.2
  Top 1.016: U$1.VDD 117.47,26.65 C16.1 83.19,26.65 | 45.09,24.11 U$3.VDD | R4.2 R14.2 42.55,44.43 38.1,39.98 R20.2 | U$6.VDD 19.68,33 23.5,36.81 C19.1 | U$2.VDD 83.19,26.65 | 83.19,26.65 C17.1 47.62,26.65 45.09,24.11 | C18.1 45.09,24.11 | R11.2 107.31,44.43 C21.+ | C20.1 KIT1.VOUT
  Bottom 0.254: 92.08,100.95 97.16,95.87 R21.2 | 92.08,100.95 81.92,100.95 71.75,90.79 R32.1 | 92.08,100.95 92.08,111.74 | 92.08,111.74 JP14.4 | 92.08,111.74 95.89,115.55 95.89,120.63 95.25,121.27 93.98,121.27 92.08,123.17 X9.1
  Bottom 1.016: R4.2 75.56,44.43 | 75.56,44.43 R11.2 | R20.2 33.66,40.62 25.4,40.62 C19.1 | C21.+ KIT1.VOUT | C17.1 75.56,44.43
+5V
  Top 0.254: 123.83,123.17 X8.1 | 79.38,123.17 X13.1
  Top 0.813: JP10.4 123.83,120 | 123.83,120 123.83,123.17 | C22.1 IC1.3 79.38,104.76 JP2.1 79.38,123.17 | 123.83,120 113.03,120 R7.2 R8.2 R30.2
  Top 1.27: C8.1 U$5.VO 22.23,87.61 | J28.1 22.23,87.61 | JP2.1 30.48,117.45 24.77,111.74 24.77,90.15 22.23,87.61
  Bottom 0.813: 107.31,86.98 KIT1.VIN | 107.31,86.98 90.81,86.98 87,90.79 C22.1 | 107.31,86.98 107.31,109.2 R30.2
/ENABLE  (via drill 0.6)
  Top 0.254: KIT1.7 94.61,61.57 85.72,52.68 85.72,49.51 v93.98,40.62
  Top 0.305: U$1.EN 130.18,29.19 113.03,29.19 110.49,31.73 U$2.EN 95.89,29.19 80.01,29.19 75.56,34.27 LED2.K 62.87,29.19 60.33,29.19 | 60.33,29.19 U$3.EN | 60.33,29.19 40.01,29.19 37.47,26.65 37.47,19.66 35.56,17.76 U$6.EN
  Bottom 0.254: v93.98,40.62 99.69,34.9 99.69,33 U$2.EN
  Bottom 0.305: J36C.1 24.26,24.62 U$6.EN | J26C.1 53.47,24.87 U$3.EN | J20C.1 91.57,24.87 U$2.EN | J13C.1 125.86,24.87 U$1.EN
ANALOG_IN
  Top 0.254: 64.14,76.81 KIT1.19 | 64.14,76.81 71.75,84.44 74.3,84.44 79.38,89.52 85.72,89.52 97.16,100.95 R33.1 R12.2 99.69,109.2 C5.1 | R10.1 57.78,73.01 61.59,76.81 64.14,76.81
ANALOG_OUT
  Top 0.254: R34.1 KIT1.18
AUX1
  Top 0.254: 12.06,97.77 X12.2
  Top 0.813: T1.C 13.97,109.2 J27.2 8.26,101.58 12.06,97.77
AUX2
  Top 0.254: 12.06,95.23 X12.3
  Top 0.813: J27.3 12.06,95.23 T2.C
CANH
  Top 0.254: IC1.7 84.45,111.11 R1.2 JP2.2 81.92,123.17 X13.2
CANL
  Top 0.254: IC1.6 87,111.11 R1.1 JP2.3 84.45,123.17 X13.3
D+
  Top 0.254: KIT1.D+ 103.5,67.92 139.06,67.92 X1.3
D-
  Top 0.254: KIT1.D- 104.14,66.02 139.06,66.02 X1.2
DIR_FEED  (via drill 0.6)
  Top 0.305: J42.3 29.84,90.79 v52.7,67.92
  Bottom 0.254: J36A.1 26.04,30.46 U$6.DIR 48.26,35.54 KIT1.22 | OK2.2 57.78,104.12 35.56,104.12 31.11,99.67 J42.3
  Bottom 0.305: KIT1.22 64.14,56.49 v52.7,67.92
DIR_X
  Top 0.254: U$1.DIR 113.03,31.73 106.68,38.08 88.9,38.08 KIT1.27
  Bottom 0.305: J13A.1 120.02,25.38 114.94,30.46 U$1.DIR
DIR_Y
  Top 0.254: U$2.DIR 80.64,42.52 KIT1.25
  Bottom 0.305: U$2.DIR 80.64,29.95 J20A.1
DIR_Z
  Top 0.254: U$3.DIR 53.34,42.52 64.14,42.52 66.67,45.06 KIT1.23
  Bottom 0.305: U$3.DIR 42.55,30.46 47.62,25.38 J26A.1
EXHAUST_ENABLE_C
  Top 0.254: JP37.4 OK2.16
  Bottom 0.254: JP37.4 56.52,119.36 53.34,122.54 X10.4
EXHAUST_ENABLE_E
  Top 0.254: JP37.3 OK2.15
  Bottom 0.254: JP37.3 59.05,119.36 55.88,122.54 X10.3
GND  (via drill 0.6)
  Top 0.254: 103.5,88.25 U4.6 | 103.5,95.87 U4.3 | 123.19,95.87 U11.3 | 123.83,88.25 U11.6 | 129.54,79.99 U11.14
  Top 0.813: 123.83,88.25 106.05,88.25 103.5,88.25 | 123.19,95.87 v105.41,95.87 103.5,95.87 | U4.14 108.58,79.36 108.58,75.55 KIT1.GND 123.83,74.28 129.54,79.99 | U11.6 124.46,88.25 125.73,88.25 129.54,84.44 129.54,79.99 | 129.54,79.99 128.91,79.99 U11.14
  Top 1.016: 106.05,88.25 v105.41,88.25
  Bottom 0.254: v105.41,95.87 105.41,89.52
  Bottom 1.016: v105.41,88.25 105.41,89.52
  pour Bottom (isolate 0.406): 1.91,125.08 149.22,125.08 149.22,1.25 1.91,1.25
LASER_ENABLE_C
  Top 0.254: JP37.2 OK2.14
  Bottom 0.254: JP37.2 61.59,119.36 58.42,122.54 X10.2
LASER_ENABLE_E
  Top 0.254: JP37.1 OK2.13
  Bottom 0.254: JP37.1 64.14,119.36 60.96,122.54 X10.1
LASER_ON  (via drill 0.6)
  Top 0.254: OK2.8 74.3,92.69 v75.56,91.42
  Bottom 0.254: KIT1.5 94.61,79.36 81.92,79.36 76.83,84.44 76.83,90.15 v75.56,91.42 | J41.1 36.83,105.39 71.75,105.39 OK2.8
LASER_ON_E
  Top 0.254: JP39.1 OK2.9
  Bottom 0.254: JP39.1 74.3,122.54 X11.1
LASER_PWM  (via drill 0.6)
  Top 0.254: v74.3,90.15 69.22,95.23 OK2.6
  Bottom 0.254: J42.1 67.31,104.76 OK2.6 | v74.3,90.15 76.2,88.25 76.2,83.8 81.28,78.72 92.71,78.72 KIT1.6
LASER_PWM_C
  Top 0.254: JP39.4 OK2.12
  Bottom 0.254: JP39.4 66.67,122.54 X11.4
LASER_PWM_E
  Top 0.254: JP39.3 OK2.11
  Bottom 0.254: JP39.3 69.22,122.54 X11.3
N$1
  Bottom 0.254: 93.34,12.68 X3.1
  Bottom 1.016: YMOT.5 99.69,11.41 98.42,12.68 | 98.42,12.68 J15.1 | 98.42,12.68 93.34,12.68 U$2.2B
N$2
  Top 0.254: 90.81,12.68 X3.2
  Top 1.016: 90.81,12.68 90.81,8.87 YMOT.4
  Bottom 0.254: 90.81,12.68 X3.2
  Bottom 0.305: U$2.2A J20C.2
  Bottom 1.016: U$2.2A 90.81,12.68
N$3
  Top 1.016: YMOT.3 88.27,11.41 X3.3
  Bottom 0.305: U$2.1A J20B.2
  Bottom 1.016: U$2.1A X3.3
N$4
  Top 0.254: 85.72,12.68 X3.4
  Top 1.016: YMOT.2 80.64,7.6 85.72,12.68
  Bottom 0.254: 85.72,12.68 X3.4
  Bottom 0.305: U$2.1B J20A.2
  Bottom 1.016: 85.72,12.68 U$2.1B
N$5
  Bottom 0.254: 127.64,12.68 X2.1
  Bottom 1.016: 132.72,12.68 XMOT.5 | U$1.2B 127.64,12.68 132.72,12.68 | 132.72,12.68 J6.1
N$6
  Top 0.254: 125.09,12.68 X2.2
  Top 1.016: 125.09,12.68 XMOT.4
  Bottom 0.254: 125.09,12.68 X2.2
  Bottom 0.305: U$1.2A J13C.2
  Bottom 1.016: 125.09,12.68 U$1.2A
N$7
  Top 1.016: XMOT.3 X2.3
  Bottom 0.305: U$1.1A J13B.2
  Bottom 1.016: X2.3 U$1.1A
N$8
  Top 0.254: 120.02,12.68 X2.4
  Top 1.016: 120.02,12.68 XMOT.2
  Bottom 0.254: 120.02,12.68 X2.4
  Bottom 0.305: U$1.1B J13A.2
  Bottom 1.016: 120.02,12.68 U$1.1B
N$9
  Bottom 0.254: 55.24,12.68 X4.1
  Bottom 1.016: ZMOT.5 60.33,12.68 | 60.33,12.68 J21.1 | U$3.2B 55.24,12.68 60.33,12.68
N$10
  Top 0.254: 52.7,12.68 X4.2
  Top 1.016: ZMOT.4 52.7,12.68
  Bottom 0.254: 52.7,12.68 X4.2
  Bottom 0.305: U$3.2A J26C.2
  Bottom 1.016: 52.7,12.68 U$3.2A
N$11
  Top 1.016: ZMOT.3 X4.3
  Bottom 0.305: U$3.1A J26B.2
  Bottom 1.016: U$3.1A X4.3
N$12
  Top 0.254: 47.62,12.68 X4.4
  Top 1.016: ZMOT.2 40.64,10.78 45.72,10.78 47.62,12.68
  Bottom 0.254: 47.62,12.68 X4.4
  Bottom 0.305: U$3.1B J26A.2
  Bottom 1.016: U$3.1B 47.62,12.68
N$13
  Top 0.254: OK2.1 R28.2
N$14
  Top 0.254: OK2.3 R29.2
N$15
  Top 0.254: OK2.5 R31.2
N$16
  Top 0.254: OK2.7 R32.2
N$17
  Top 0.254: OK1.2 51.44,98.41 R23.2
N$18
  Top 0.254: R24.2 OK1.4
N$19
  Top 0.254: OK1.6 41.27,98.41 R26.2
N$20
  Top 0.254: R27.2 OK1.8
N$22
  Bottom 1.016: X2.5 116.2,12.68 111.12,7.6 XMOT.1 110.49,7.6 J12.1
N$23
  Bottom 1.016: 73.03,7.6 78.11,12.68 X3.5 | YMOT.1 73.03,7.6 | 73.03,7.6 J19.1
N$24
  Bottom 1.016: 33.02,7.6 38.1,12.68 X4.5
  Bottom 1.27: ZMOT.1 33.02,7.6 J25.1
N$28
  Bottom 0.254: KIT1.VU 119.38,63.48 X1.1
N$29
  Top 0.254: J7.6 R6.1 | J7.2 122.56,36.81 120.02,34.27 U$1.SLP
  Top 0.305: U$1.SLP U$1.RST | J7.2 J7.4 J7.6
N$30
  Top 0.305: U$1.MS1 J7.5
N$31
  Top 0.305: U$1.MS2 J7.3
N$32
  Top 0.305: R9.2 J7.1 U$1.MS3
N$34
  Top 0.254: U$2.SLP 85.72,34.27 88.27,36.81 J16.2
  Top 0.305: U$2.SLP U$2.RST | R11.1 J16.6 J16.4 J16.2
N$35
  Top 0.305: U$2.MS1 J16.5
N$36
  Top 0.305: U$2.MS2 J16.3
N$37
  Top 0.305: U$2.MS3 J16.1 R13.2
N$39
  Top 0.254: J22.2 50.16,36.81 47.62,34.27 U$3.SLP
  Top 0.305: U$3.SLP U$3.RST | R14.1 J22.6 J22.4 J22.2
N$40
  Top 0.305: U$3.MS1 J22.5
N$41
  Top 0.305: U$3.MS2 J22.3
N$42
  Top 0.305: R16.2 J22.1 U$3.MS3
N$49
  Top 0.254: R33.2 JP14.2 97.16,123.17 X9.3
N$55
  Bottom 1.016: J35.1 8.26,45.06 | MOT_FEED.1 8.26,45.06 | 8.26,45.06 13.34,39.98 X5.5
N$57
  Top 0.254: R2.2 128.27,41.89 J4.A1
N$60
  Top 0.254: JP14.3 94.61,123.17 X9.2
  Bottom 0.254: R34.2 81.92,102.22 89.53,102.22 90.81,103.48 90.81,119.36 91.44,120 93.98,120 94.61,119.36 JP14.3
N$64
  Top 0.254: T1.B 19.68,114.92 R15.1
N$65
  Top 0.254: T2.B 19.68,99.67 R17.1
N$68
  Top 0.254: JP39.2 OK2.10
  Bottom 0.254: JP39.2 71.75,122.54 X11.2
N$75
  Bottom 0.254: R3.2 125.73,47.6 128.27,50.14 J4.A2
N$76
  Bottom 0.254: R15.2 27.3,111.11 28.57,109.84 J41.2
N$77
  Top 0.254: R17.2 J42.2
N$82
  Top 0.254: 13.34,22.84 X5.1
  Top 1.016: U$6.2B 13.34,22.84 MOT_FEED.5
  Bottom 0.813: MOT_FEED.5 J30.1
N$83
  Top 0.254: 12.7,25.38 X5.2
  Top 1.016: MOT_FEED.4 12.7,25.38 U$6.2A
  Bottom 0.305: U$6.2A J36C.2
N$84
  Top 1.016: U$6.1A X5.3 8.26,32.36 MOT_FEED.3
  Bottom 0.305: U$6.1A J36B.2
N$85
  Top 0.254: 13.34,30.46 X5.4
  Top 1.016: U$6.1B 15.88,30.46 | 15.88,30.46 13.34,30.46 | 15.88,30.46 15.88,33 MOT_FEED.2
  Bottom 0.305: U$6.1B J36A.2
N$86
  Bottom 0.254: LED3.A R30.1
N$90
  Top 0.254: J31.2 R20.1 33.66,30.46 U$6.SLP
  Top 0.305: U$6.RST U$6.SLP | J31.6 J31.4 J31.2
N$91
  Top 0.305: U$6.MS1 J31.5
N$92
  Top 0.305: U$6.MS2 J31.3
N$93
  Top 0.305: U$6.MS3 J31.1 R25.2
N$105
  Top 0.406: LED1.A 143.51,36.81 R5.1
N$106
  Top 0.305: R4.1 LED2.A
P8  (via drill 0.6)
  Top 0.254: v81.92,90.79 76.2,96.5 76.2,104.12 75.56,104.76 56.52,104.76 55.24,103.48 55.24,95.23 52.07,92.06 46.35,92.06 OK1.12 | KIT1.8 92.08,78.09 R21.1
  Bottom 0.254: R21.1 89.53,83.17 v81.92,90.79
P11
  Top 0.254: U11.2 122.56,98.41 103.5,98.41 U4.2 102.87,98.41 97.16,98.41 90.81,92.06 90.81,86.34 84.45,79.99 KIT1.11
P12
  Top 0.254: KIT1.12 83.82,72.37 89.53,72.37 90.81,73.64 90.81,78.72 97.79,85.7 102.23,85.7 U4.7 102.87,85.7 123.83,85.7 U11.7
P13  (via drill 0.6)
  Top 0.254: v88.27,75.55 88.27,77.45 101.6,90.79 102.87,90.79 U4.5 103.5,90.79 123.83,90.79 U11.5
  Bottom 0.254: v88.27,75.55 80.64,75.55 KIT1.13
P14
  Top 0.254: U11.1 124.46,100.95 103.5,100.95 U4.1 102.87,100.95 98.42,100.95 88.27,90.79 88.27,86.34 76.83,74.91 KIT1.14
P15
  Top 0.254: R18.1 KIT1.15
  Bottom 0.254: OK1.16 53.98,85.7 59.69,79.99 71.12,79.99 R18.1
P16
  Top 0.254: R19.1 KIT1.16
  Bottom 0.254: OK1.14 59.05,79.36 69.22,79.36 R19.1
P17
  Top 0.254: KIT1.17 R22.1
  Bottom 0.254: OK1.10 49.53,78.72 67.31,78.72 R22.1
P29  (via drill 0.6)
  Top 0.254: KIT1.29 80.64,52.68 80.64,67.92 75.56,73.01 75.56,75.55 79.38,79.36 v79.38,86.98
  Bottom 0.254: IC1.1 79.38,94.59 v79.38,86.98
P30  (via drill 0.6)
  Top 0.254: KIT1.30 84.45,69.2 80.64,73.01 80.64,77.45 89.53,86.34 v89.53,90.15
  Bottom 0.254: IC1.4 v89.53,90.15
RD+
  Top 0.254: J4.4 137.16,48.24 138.43,46.97 138.43,43.16 135.25,39.98 122.56,39.98 113.03,49.51 99.06,49.51 KIT1.RD+
RD-
  Top 0.254: J4.6 132.08,45.7 131.44,46.33 117.47,46.33 113.67,50.14 100.97,50.14 KIT1.RD-
SCL
  Top 0.254: KIT1.10 87,78.09 100.97,92.06 125.09,92.06 132.08,99.04 132.08,111.74 128.91,114.92 | 128.91,114.92 JP10.2 128.91,123.17 X8.3 | 128.91,114.92 R8.1
SDA
  Top 0.254: JP10.3 126.36,123.17 X8.2
  Bottom 0.254: KIT1.9 90.81,73.01 111.12,73.01 112.39,74.28 112.39,109.2 R7.1 126.36,123.17 X8.2
STEP_FEED
  Top 0.254: U$6.STEP 34.92,36.81 34.92,39.35 46.99,51.41 53.98,51.41 | 53.98,51.41 KIT1.21 | 53.98,85.7 53.98,51.41 | OK2.4 64.14,99.67 55.24,90.79 55.24,86.98 53.98,85.7 | 53.98,85.7 36.2,85.7 33.66,88.25 33.66,103.48 J41.3
  Bottom 0.254: U$6.STEP 26.04,27.92 J36B.1
STEP_X
  Top 0.254: U$1.STEP 109.86,39.35 90.81,39.35 KIT1.28
  Bottom 0.305: J13B.1 122.56,25.38 117.47,30.46 U$1.STEP
STEP_Y
  Top 0.254: U$2.STEP 83.19,42.52 KIT1.26
  Bottom 0.305: U$2.STEP 83.19,29.95 J20B.1
STEP_Z
  Top 0.254: KIT1.20 61.59,59.03 KIT1.24
  Bottom 0.254: KIT1.24 67.94,50.14 64.14,50.14 48.26,34.27 47.62,34.27 U$3.STEP
  Bottom 0.305: U$3.STEP 45.09,30.46 50.16,25.38 J26B.1
TD+
  Top 0.254: KIT1.TD+ 95.25,54.59 130.81,54.59 133.35,52.05 J4.1
TD-
  Top 0.254: KIT1.TD- 95.89,52.68 123.83,52.68 127.64,48.88 129.54,48.88 130.18,49.51 J4.3
V_ENDSTOP
  Top 0.406: JP29.4 51.44,111.11 48.9,108.56 43.81,108.56 | JP34.4 41.27,111.11 43.81,108.56 | 43.81,108.56 OK1.5 43.81,95.87 | 43.81,95.87 40.01,95.87 OK1.7 | 48.9,95.87 OK1.3 | 43.81,95.87 48.9,95.87 | 48.9,95.87 52.7,95.87 OK1.1
  Top 0.813: 12.06,87.61 X12.4
  Top 1.27: J27.4 12.06,87.61 14.61,85.07 J28.2
  Bottom 0.254: JP34.4 41.27,115.55 34.29,122.54 X7.1 | JP29.4 51.44,118.73 47.62,122.54 X6.1
  Bottom 0.406: J28.2 27.94,85.07 38.73,95.87 OK1.7
VAA
  Top 1.27: C6.+ U$5.VI C7.1
  Bottom 1.27: C6.+ 10.16,69.2 POWER.2 J40.1
VMOT
  Top 0.254: R10.2 34.92,67.92 25.72,58.72
  Top 0.406: R5.2 C11.+
  Top 1.27: 98.42,15.86 U$2.VMOT | 60.33,15.86 U$3.VMOT | 12.06,79.36 15.24,82.53 J28.3
  Top 1.93: C2.+ C15.1 | 27.3,13.32 18.41,13.32
  Top 2.184: 105.41,15.86 98.42,15.86 66.67,15.86 | C2.+ 18.41,13.32 U$6.VMOT | C9.+ C14.1 66.67,15.86 | POWER.1 12.06,79.36 12.06,72.37 25.72,58.72 C3.1 C4.+ 27.3,13.32 36.2,13.32 38.73,15.86 60.33,15.86 66.67,15.86 | C11.+ C12.1 U$1.VMOT 132.72,17.12 131.44,15.86 105.41,15.86 | C10.+ C13.1 105.41,15.86
  Bottom 1.016: U$3.VMOT J21.2 | U$6.VMOT J30.2 | U$2.VMOT J15.2
  Bottom 1.27: U$1.VMOT J6.2 | POWER.1 J40.2
X_HOME
  Top 0.254: R23.1 JP29.3
  Bottom 0.254: JP29.3 48.9,118.73 45.09,122.54 X6.2
Y_HOME
  Top 0.254: R24.1 JP29.2
  Bottom 0.254: JP29.2 46.35,118.73 42.55,122.54 X6.3
Z+
  Top 0.254: R26.1 JP34.3
  Bottom 0.254: JP34.3 38.73,115.55 31.75,122.54 X7.2
Z-
  Top 0.254: R27.1 JP34.2
  Bottom 0.254: JP34.2 36.2,115.55 29.21,122.54 X7.3

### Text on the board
tNames: ANALOG | I2C | AUX
tValues: Y_Home | X_Home | LASER | EXHAUST | Z- | Z+ | ON | PWM | ENA | ENA | GND | O2 | O1 | V_End | +5V | V_Endstop | Vmot | LAOS #42 V1.0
